(* Logix 5000 AddOnInstructionDefinition export AMCI_ANG1E_Absolute_Encoder_Move; software revision 20.03 *)

ADD_ON_INSTRUCTION AMCI_ANG1E_Absolute_Encoder_Move   (* revision 5.0, vendor AMCI, ExecuteEnableInFalse *)
// Revision note:
// Version 5.0 added the (hidden) ability to program the motor current and unlatched the error bit if the rung goes false.
VAR_INPUT
   Axis_Status_Bits : INT; {required}
   slot_axis_number : INT; {required}
   Type_0_for_standard_1_for_indexed : BOOL;
   Target_Position : DINT; {required}
   Programmed_Speed : DINT; {required}
   Acceleration : INT; {required}
   Deceleration : INT; {required}
   motor_current : INT;
   Jerk : INT;
END_VAR
VAR_IN_OUT
   AMCI_ANG1E_output_data : INT[10]; {required}
END_VAR
VAR_OUTPUT
   EN : BOOL; {access Read Only, visible}
   ER : BOOL; {access Read Only, visible}
END_VAR
VAR
   Upper_Result_X_1000 : DINT;
   command_data_block : INT[10];
        [0]   // Command Bits MSW
        [1]   // Command Bits LSW
        [2]   // Upper Target Position
        [3]   // Lower Target Position
        [4]   // Upper Programmed Speed
        [5]   // Lower Programmed Speed
   index : INT;
END_VAR

ROUTINE EnableInFalse   (* ladder *)
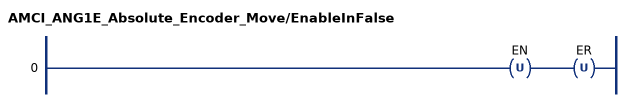
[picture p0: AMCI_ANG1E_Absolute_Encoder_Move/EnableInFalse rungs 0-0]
   0: OTU(EN)OTU(ER);
END_ROUTINE

ROUTINE Logic   (* ladder *)
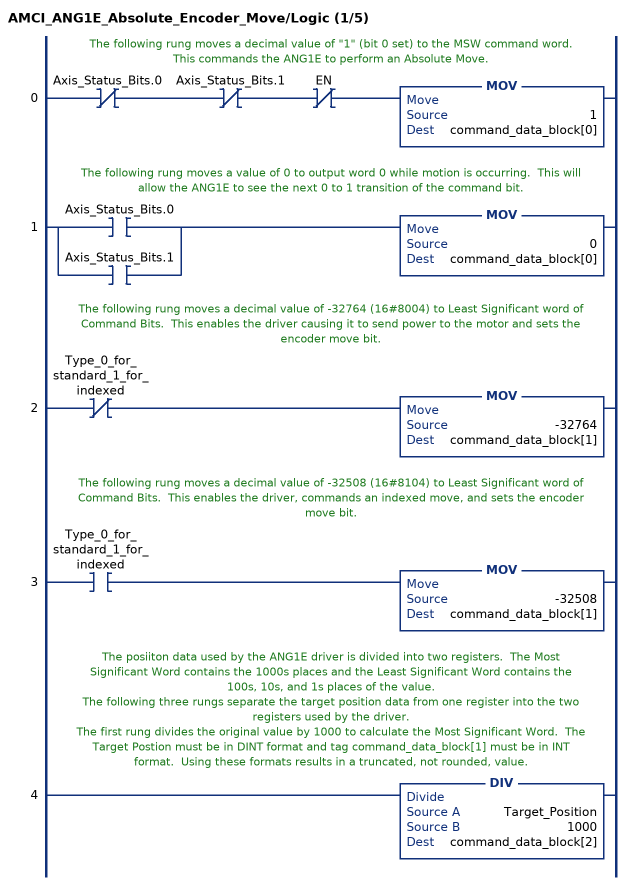
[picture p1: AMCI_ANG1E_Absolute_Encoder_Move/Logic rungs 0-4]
   // The following rung moves a decimal value of "1" (bit 0 set) to the MSW command word.  This commands the ANG1E to perform an Absolute Move.
   0: XIO(Axis_Status_Bits.0)XIO(Axis_Status_Bits.1)XIO(EN)MOV(1,command_data_block[0]);
   // The following rung moves a value of 0 to output word 0 while motion is occurring.  This will allow the ANG1E to see the next 0 to 1 transition of the command bit.
   1: [XIC(Axis_Status_Bits.0) ,XIC(Axis_Status_Bits.1) ]MOV(0,command_data_block[0]);
   // The following rung moves a decimal value of -32764 (16#8004) to Least Significant word of Command Bits.  This enables the driver causing it to send power to the motor and sets the encoder move bit.
   2: XIO(Type_0_for_standard_1_for_indexed)MOV(-32764,command_data_block[1]);
   // The following rung moves a decimal value of -32508 (16#8104) to Least Significant word of Command Bits.  This enables the driver, commands an indexed move, and sets the encoder move bit.
   3: XIC(Type_0_for_standard_1_for_indexed)MOV(-32508,command_data_block[1]);
   // The posiiton data used by the ANG1E driver is divided into two registers.  The Most Significant Word contains the 1000s places and the Least Significant Word contains the 100s, 10s, and 1s places of the value.
   // The following three rungs separate the target position data from one register into the two registers used by the driver.
   // The first rung divides the original value by 1000 to calculate the Most Significant Word.  The Target Postion must be in DINT format and tag command_data_block[1] must be in INT format.  Using these formats results in a truncated, not rounded, value.
   4: DIV(Target_Position,1000,command_data_block[2]);
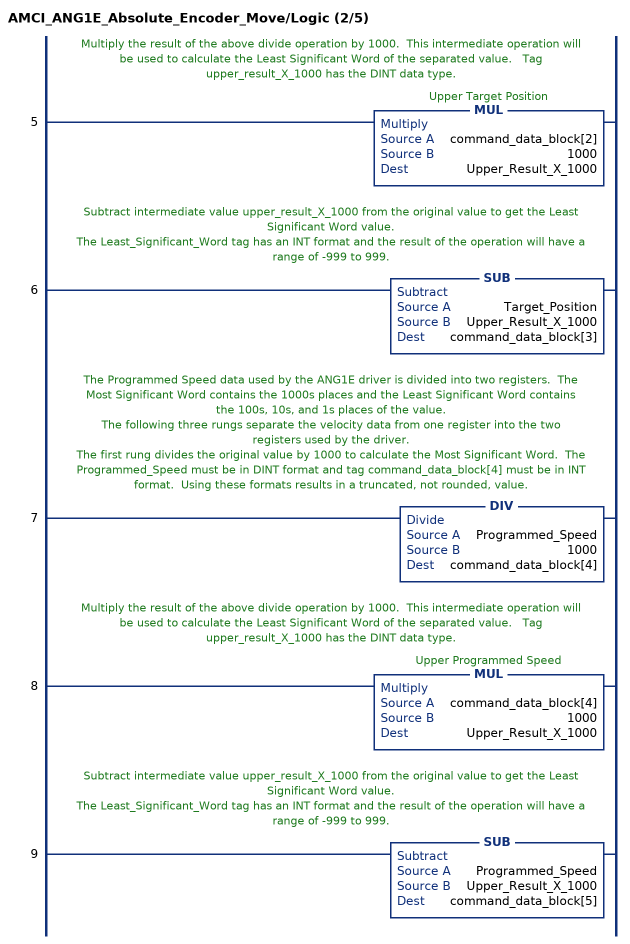
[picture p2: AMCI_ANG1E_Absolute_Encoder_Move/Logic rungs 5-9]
   // Multiply the result of the above divide operation by 1000.  This intermediate operation will be used to calculate the Least Significant Word of the separated value.   Tag upper_result_X_1000 has the DINT data type.
   5: MUL(command_data_block[2],1000,Upper_Result_X_1000);
   // Subtract intermediate value upper_result_X_1000 from the original value to get the Least Significant Word value.
   // The Least_Significant_Word tag has an INT format and the result of the operation will have a range of -999 to 999.
   6: SUB(Target_Position,Upper_Result_X_1000,command_data_block[3]);
   // The Programmed Speed data used by the ANG1E driver is divided into two registers.  The Most Significant Word contains the 1000s places and the Least Significant Word contains the 100s, 10s, and 1s places of the value.
   // The following three rungs separate the velocity data from one register into the two registers used by the driver.
   // The first rung divides the original value by 1000 to calculate the Most Significant Word.  The Programmed_Speed must be in DINT format and tag command_data_block[4] must be in INT format.  Using these formats results in a truncated, not rounded, value.
   7: DIV(Programmed_Speed,1000,command_data_block[4]);
   // Multiply the result of the above divide operation by 1000.  This intermediate operation will be used to calculate the Least Significant Word of the separated value.   Tag upper_result_X_1000 has the DINT data type.
   8: MUL(command_data_block[4],1000,Upper_Result_X_1000);
   // Subtract intermediate value upper_result_X_1000 from the original value to get the Least Significant Word value.
   // The Least_Significant_Word tag has an INT format and the result of the operation will have a range of -999 to 999.
   9: SUB(Programmed_Speed,Upper_Result_X_1000,command_data_block[5]);
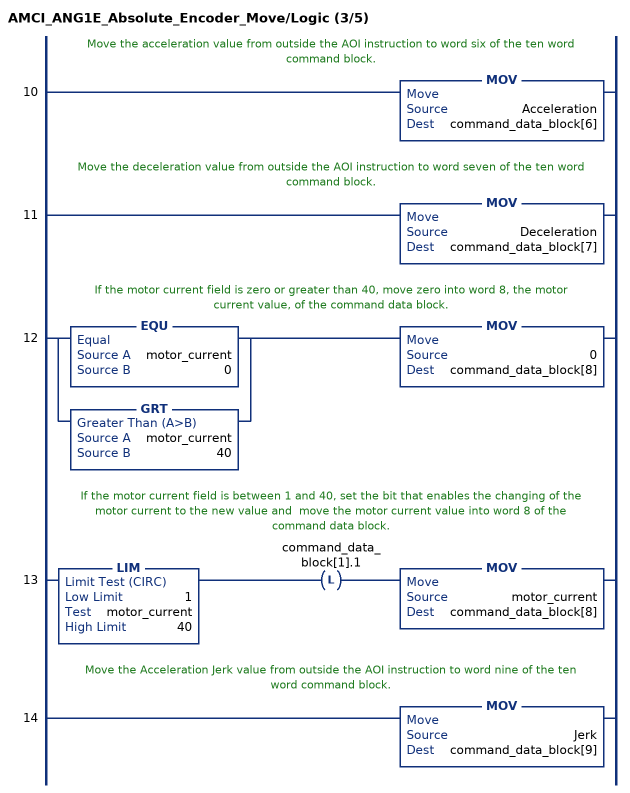
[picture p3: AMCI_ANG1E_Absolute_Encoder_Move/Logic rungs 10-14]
   // Move the acceleration value from outside the AOI instruction to word six of the ten word command block.
   10: MOV(Acceleration,command_data_block[6]);
   // Move the deceleration value from outside the AOI instruction to word seven of the ten word command block.
   11: MOV(Deceleration,command_data_block[7]);
   // If the motor current field is zero or greater than 40, move zero into word 8, the motor current value, of the command data block.
   12: [EQU(motor_current,0) ,GRT(motor_current,40) ]MOV(0,command_data_block[8]);
   // If the motor current field is between 1 and 40, set the bit that enables the changing of the motor current to the new value and  move the motor current value into word 8 of the command data block.
   13: LIM(1,motor_current,40)OTL(command_data_block[1].1)MOV(motor_current,command_data_block[8]);
   // Move the Acceleration Jerk value from outside the AOI instruction to word nine of the ten word command block.
   14: MOV(Jerk,command_data_block[9]);
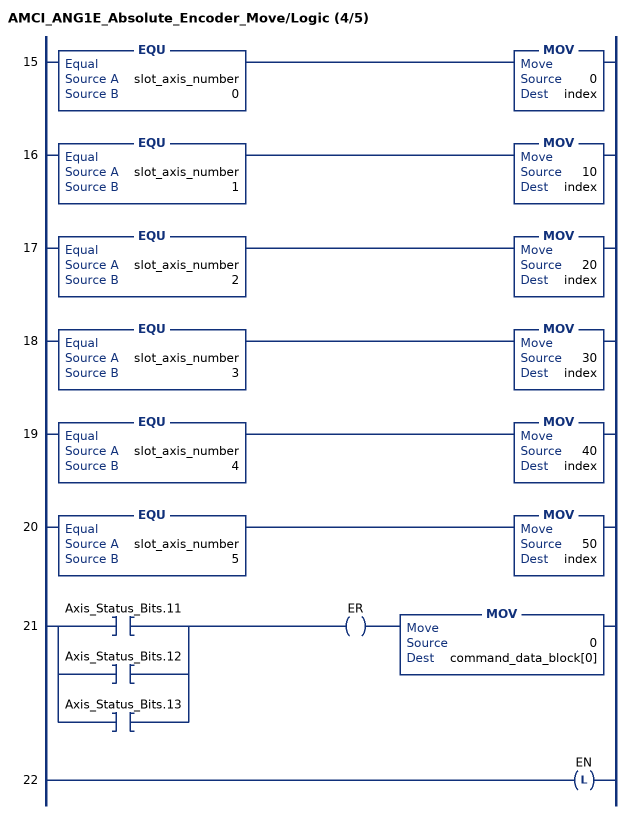
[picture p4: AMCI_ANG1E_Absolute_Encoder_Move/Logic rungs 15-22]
   15: EQU(slot_axis_number,0)MOV(0,index);
   16: EQU(slot_axis_number,1)MOV(10,index);
   17: EQU(slot_axis_number,2)MOV(20,index);
   18: EQU(slot_axis_number,3)MOV(30,index);
   19: EQU(slot_axis_number,4)MOV(40,index);
   20: EQU(slot_axis_number,5)MOV(50,index);
   21: [XIC(Axis_Status_Bits.11) ,XIC(Axis_Status_Bits.12) ,XIC(Axis_Status_Bits.13) ]OTE(ER)MOV(0,command_data_block[0]);
   22: OTL(EN);
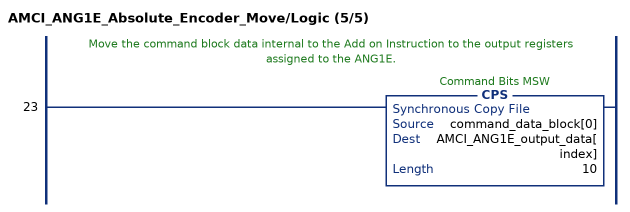
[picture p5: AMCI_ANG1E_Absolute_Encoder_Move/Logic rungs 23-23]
   // Move the command block data internal to the Add on Instruction to the output registers assigned to the ANG1E.
   23: CPS(command_data_block[0],AMCI_ANG1E_output_data[index],10);
END_ROUTINE
END_ADD_ON_INSTRUCTION
